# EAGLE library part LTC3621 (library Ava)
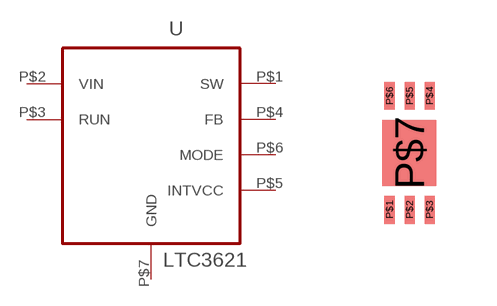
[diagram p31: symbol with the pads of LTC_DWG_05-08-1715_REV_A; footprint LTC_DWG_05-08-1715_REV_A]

Designator prefix -

## LTC3621  [LTC_DWG_05-08-1715_REV_A]
P$1  SW  out
P$2  VIN  pwr
P$3  RUN  pas
P$4  FB  in
P$5  INTVCC  pas
P$6  MODE  in
P$7  GND  pas

## Footprint LTC_DWG_05-08-1715_REV_A (pad centres in mm)
smd 0.25 x 0.7: P$1 -0.5,-1.425; P$2 0,-1.425; P$3 0.5,-1.425; P$4 0.5,1.425; P$5 0,1.425; P$6 -0.5,1.425
smd 1.35 x 1.65: P$7 0,0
